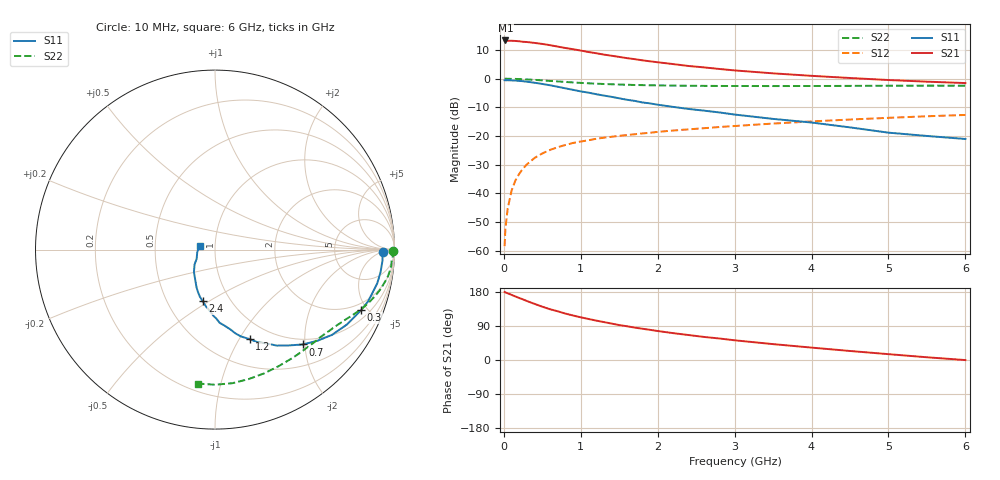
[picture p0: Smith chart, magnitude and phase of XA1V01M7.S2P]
! SIEMENS Discrete & RF Semiconductors
! BFY180
! Si NPN RF Bipolar Junction Transistor in MICRO-X
! VCE = 1 V  IC = 1.7 mA
! Common Emitter S-Parameters:  May  1997
# GHz  S  MA  R  50
!  f  S11  S21  S12  S22
! GHz  MAG  ANG  MAG  ANG  MAG  ANG  MAG  ANG
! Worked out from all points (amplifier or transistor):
!   36 points, 10 MHz to 6 GHz, reference 50 ohm
!   highest |S21| = 13.3 dB at 20 MHz (marker M1)
!   |S21| within 3 dB of that: start of sweep to 887.9 MHz
!   unconditionally stable (mu >= 1): 1.983 GHz to end of sweep
!   at 250 MHz: K = 0.16, MSG = 22.1 dB, |S12| = -31.3 dB
!   at 1.4 GHz: K = 0.82, MSG = 14.1 dB, |S12| = -20.3 dB
!   at 6 GHz: K = 1.17, MAG = 3.1 dB, |S12| = -12.7 dB
!   S11 on the Smith chart (normalised r, x): 10 MHz: 29, -6; 300 MHz: 1.51, -4.57; 700 MHz: 0.89, -1.96; 1.2 GHz: 0.79, -1.11; 2.4 GHz: 0.74, -0.47; 6 GHz: 0.84, +0.04
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0.01  0.9355 -0.8  4.536 179.4  0.0012 85.0  0.9922 -0.3
0.02  0.9336 -1.6  4.615 178.3  0.0024 88.2  0.9943 -0.7
0.05  0.9352 -3.8  4.554 176.0  0.0054 86.3  0.9928 -1.8
0.1  0.9309 -7.7  4.555 171.9  0.0111 85.2  0.9862 -3.5
0.2  0.9099 -15.3  4.469 163.6  0.0219 80.5  0.981 -7.0
0.3  0.8816 -22.4  4.334 155.6  0.032 75.7  0.9669 -10.2
0.4  0.8452 -29.6  4.178 148.0  0.0414 71.8  0.95 -13.2
0.5  0.8065 -36.1  4.014 140.7  0.0495 67.0  0.93 -16.0
0.6  0.7639 -41.7  3.821 134.0  0.057 64.1  0.9104 -18.5
0.7  0.7203 -47.2  3.607 128.6  0.0636 60.9  0.8921 -20.7
0.9  0.6365 -57.2  3.248 117.4  0.0755 55.7  0.8558 -24.7
1.1  0.5683 -65.3  2.902 108.3  0.0841 52.0  0.8265 -28.0
1.2  0.5344 -68.9  2.767 104.0  0.0892 50.4  0.8152 -29.6
1.5  0.4528 -79.1  2.385 92.2  0.1004 46.8  0.787 -34.1
1.7  0.4086 -86.4  2.181 85.5  0.1069 45.2  0.7725 -36.9
2.2  0.3211 -98.9  1.789 70.9  0.1243 40.9  0.7547 -43.9
2.4  0.2954 -103.6  1.657 65.9  0.1302 39.6  0.7494 -46.6
3  0.236 -115.7  1.387 52.0  0.149 35.3  0.742 -54.7
3.5  0.1982 -124.0  1.233 41.9  0.1644 31.9  0.74 -61.5
4.5  0.141 -143.9  1.023 23.8  0.1932 24.3  0.7454 -75.4
5.5  0.1 -171.7  0.883 7.2  0.2203 16.0  0.7529 -90.0
6  0.0885 165.1  0.835 -0.2  0.2322 11.6  0.7523 -97.3
